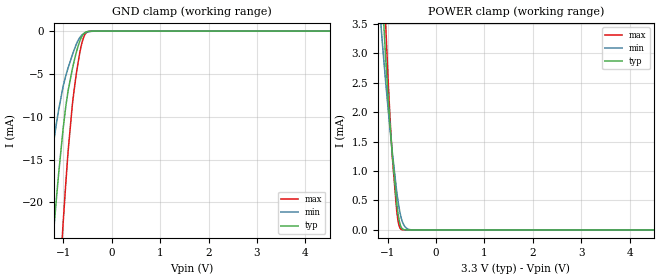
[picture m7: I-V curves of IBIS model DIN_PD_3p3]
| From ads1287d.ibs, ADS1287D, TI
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|   Model
[Model]   DIN_PD_3p3
Model_type   Input
Vinl = 0.99
Vinh = 2.31
|   typ   min   max
C_comp   2.168pF   1.862pF   2.430pF
[Voltage Range]   3.3   3   3.6
[Temperature Range]   27   125   -40
[Power Clamp Reference]   3.3   3   3.6
[GND Clamp Reference]   0   0   0
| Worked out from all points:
|   GND clamp passes 1 mA (typ) near -0.65 V on its own axis
|   POWER clamp passes 1 mA (typ) near -0.87 V on its own axis
[GND Clamp]
|   Voltage   I(typ)   I(min)   I(max)
-3.3V     -208.6mA   -142.2mA   -265.1mA
-1.459V   -42.29mA   -24.16mA   -67.13mA
-1.201V   -23.19mA   -12.84mA   -40.72mA
-1.102V   -16.77mA   -9.268mA   -31.09mA
-1.013V   -11.69mA   -6.602mA   -22.91mA
-904.2mV  -6.934mA   -4.282mA   -13.99mA
-815.1mV  -4.375mA   -2.764mA   -8.476mA
-745.8mV  -2.722mA   -1.687mA   -5.44mA
-666.6mV  -1.229mA   -790.8uA   -2.639mA
-607.2mV  -505.8uA   -405uA     -1.138mA
-537.9mV  -122.2uA   -173.5uA   -256.7uA
6.6V      0A         0A         0A
[POWER Clamp]
|   Voltage   I(typ)   I(min)   I(max)
-3.3V     45.09mA    35.55mA    54.77mA
-1.132V   4.283mA    3.402mA    5.313mA
-1.112V   3.967mA    3.196mA    4.902mA
-1.053V   3.073mA    2.614mA    3.706mA
-1.043V   2.934mA    2.522mA    3.513mA
-904.2mV  1.279mA    1.318mA    1.238mA
-805.2mV  399.6uA    602.4uA    268.4uA
-765.6mV  173.8uA    383.3uA    77.66uA
-716.1mV  39.32uA    191.4uA    8.74uA
-627mV    1.414uA    41.85uA    76.3nA
-478.5mV  0A         927nA      0A
6.6V      0A         0A         0A
